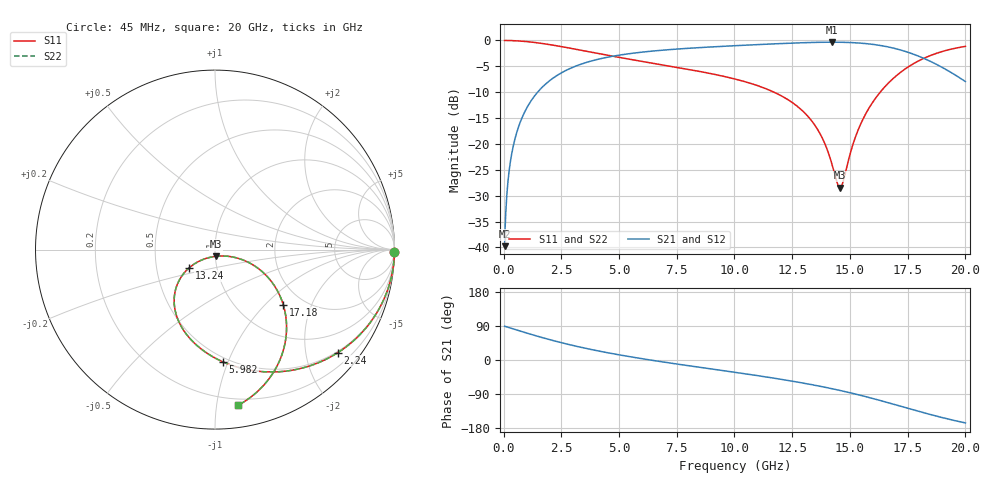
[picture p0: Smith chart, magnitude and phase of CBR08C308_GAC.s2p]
! S-parameter model data by Modelithics Inc.  support@modelithics.com 813-866-6335  Tampa FL USA
! S-Parameter data specifications:
! Substrate: 20-mil Rogers 4350B, substrate thickness, H=0.508mm, Dielectric constant, Er=3.75
! PCB Mounting Pad Footprint: Pad width, PadW=1.45mm , Pad length, PadL=1mm , Pad gap, PadG (edge-to-edge)=0.6mm , Reference planes=2.6mm apart
#  GHz  S  MA  R 50
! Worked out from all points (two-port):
!   801 points, 45 MHz to 20 GHz, reference 50 ohm
!   highest |S21| = -0.33 dB at 14.21 GHz (marker M1); lowest = -39.8 dB at 45 MHz (marker M2)
!   |S21| within 3 dB of the highest: 4.396 GHz to 18.13 GHz (13.74 GHz wide, 122 % of centre)
!   lowest |S11| = -28.5 dB at 14.56 GHz (marker M3), VSWR 1.08, Z = 50.2 - j3.78 ohm
!   |S11| at or under -10 dB: 11.71 GHz to 16.31 GHz (4.597 GHz wide, 32.8 % of centre)
!   |S22| runs from -28.5 to 0.0 dB; largest |S21 - S12| = 0
!   S11 on the Smith chart (normalised r, x): 45 MHz: open; 2.24 GHz: 0.47, -2.67; 5.982 GHz: 0.46, -0.96; 13.24 GHz: 0.73, -0.16; 17.18 GHz: 1.59, -1.29; 20 GHz: 0.15, -1.15
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0.045  0.9999 -0.9  0.01027 89.1  0.01027 89.1  0.9999 -0.9
0.194662  0.999 -3.7  0.0444 86.3  0.0444 86.3  0.999 -3.7
0.269494  0.9981 -5.1  0.0614 84.8  0.0614 84.8  0.9981 -5.1
0.419156  0.9954 -8.0  0.0952 82.0  0.0952 82.0  0.9954 -8.0
0.64365  0.9893 -12.2  0.1451 77.7  0.1451 77.7  0.9893 -12.2
1.292188  0.9592 -24.1  0.281 65.8  0.281 65.8  0.9592 -24.1
2.24005  0.893 -40.1  0.4475 49.8  0.4475 49.8  0.893 -40.1
3.387462  0.8018 -56.7  0.5934 33.0  0.5934 33.0  0.8018 -56.7
5.981612  0.628 -85.8  0.7705 3.6  0.7705 3.6  0.628 -85.8
6.704981  0.5893 -92.6  0.7991 -3.3  0.7991 -3.3  0.5893 -92.6
10.0225  0.4238 -120.5  0.89 -32.5  0.89 -32.5  0.4238 -120.5
11.96811  0.2964 -136.3  0.9324 -50.4  0.9324 -50.4  0.2964 -136.3
13.24024  0.1783 -144.8  0.9548 -63.9  0.9548 -63.9  0.1783 -144.8
13.36496  0.1647 -145.2  0.9564 -65.3  0.9564 -65.3  0.1647 -145.2
13.83889  0.1096 -143.9  0.961 -70.9  0.961 -70.9  0.1096 -143.9
14.21305  0.06465 -133.0  0.9622 -75.6  0.9622 -75.6  0.06465 -133.0
14.56226  0.03774 -85.0  0.9609 -80.3  0.9609 -80.3  0.03774 -85.0
15.51013  0.1637 -20.3  0.9401 -94.0  0.9401 -94.0  0.1637 -20.3
16.68248  0.3909 -31.6  0.8632 -113.1  0.8632 -113.1  0.3909 -31.6
17.18136  0.4899 -39.0  0.8102 -121.8  0.8102 -121.8  0.4899 -39.0
18.42854  0.7068 -58.8  0.6365 -143.0  0.6365 -143.0  0.7068 -58.8
20  0.8767 -81.5  0.4007 -166.0  0.4007 -166.0  0.8767 -81.5
